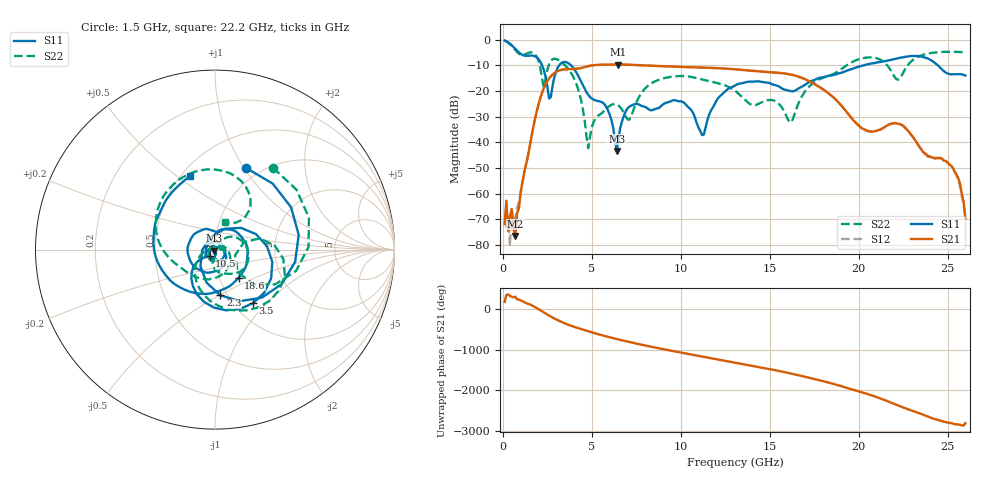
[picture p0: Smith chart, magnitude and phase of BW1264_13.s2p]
!Keysight Technologies,N5245B,MY57181159,A.13.60.06
!Date: Friday, December 18, 2020 23:52:35
!Correction: S11(Full 2 Port(1,2))
!S21(Full 2 Port(1,2))
!S12(Full 2 Port(1,2))
!S22(Full 2 Port(1,2))
!S2P File: Measurements: S11, S21, S12, S22:
# Hz S  dB  R 50
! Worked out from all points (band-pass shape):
!   260 points, 100 MHz to 26 GHz, reference 50 ohm
!   highest |S21| = -9.75 dB at 6.5 GHz (marker M1); lowest = -76.5 dB at 700 MHz (marker M2)
!   |S21| within 3 dB of the highest: 2.964 GHz to 15.03 GHz (12.07 GHz wide, 134 % of centre)
!   lowest |S11| = -43.4 dB at 6.4 GHz (marker M3), VSWR 1.01, Z = 49.6 - j0.571 ohm
!   |S11| at or under -10 dB: 2.204 GHz to 3.172 GHz (968 MHz wide, 36 % of centre); 3.827 GHz to 20.31 GHz (16.48 GHz wide, 137 % of centre); 24.44 GHz to end of sweep
!   |S22| runs from -42.3 to -0.4 dB; largest |S21 - S12| = 0.00055
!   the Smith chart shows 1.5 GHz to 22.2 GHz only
!   S11 on the Smith chart (normalised r, x): 1.5 GHz: 0.86, +1.02; 2.3 GHz: 0.93, -0.51; 3.5 GHz: 1.22, -0.84; 10.5 GHz: 0.94, -0.06; 18.6 GHz: 1.23, -0.40; 22.2 GHz: 0.56, +0.56
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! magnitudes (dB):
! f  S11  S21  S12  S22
! 100 MHz  -0.4  -71.9  -70.2  -0.4
! 400 MHz  -1.6  -69.0  -80.5  -1.8
! 700 MHz  -3.6  -76.5  -69.7  -4.1
! 1.5 GHz  -6.3  -42.1  -42.1  -5.1
! 2.3 GHz  -11.8  -19.0  -19.0  -18.7
! 2.6 GHz  -23.0  -15.2  -15.2  -9.6
! 3.5 GHz  -8.7  -11.6  -11.6  -10.1
! 4.5 GHz  -17.9  -10.9  -10.9  -27.1
! 4.8 GHz  -21.5  -10.4  -10.4  -42.3
! 6.4 GHz  -43.4  -9.8  -9.7  -25.3
! 6.5 GHz  -38.7  -9.7  -9.7  -25.7
! 8.8 GHz  -26.5  -10.3  -10.3  -15.6
! 10.5 GHz  -26.8  -10.8  -10.8  -14.5
! 11.3 GHz  -37.0  -10.9  -10.9  -15.7
! 13.1 GHz  -17.7  -11.6  -11.6  -20.2
! 16.2 GHz  -20.1  -13.7  -13.7  -32.2
! 17.4 GHz  -16.0  -16.9  -16.9  -17.2
! 18.6 GHz  -13.8  -22.6  -22.6  -13.4
! 21.7 GHz  -8.1  -33.1  -33.1  -10.9
! 22.2 GHz  -7.3  -32.8  -32.7  -15.7
! 25.3 GHz  -13.5  -50.0  -49.9  -4.8
! 26 GHz  -14.0  -69.8  -69.7  -5.0
